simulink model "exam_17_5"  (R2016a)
settings: Solver=ode15s  StartTime=0.0  StopTime=10  RelTol=1e-3
libraries: powerlib x7, dspxfrm3 x2

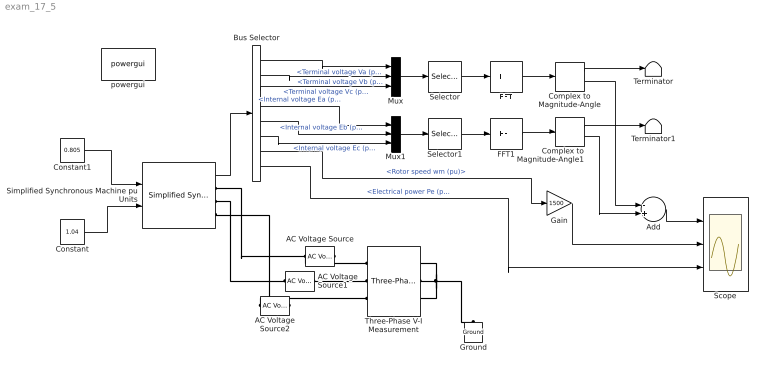
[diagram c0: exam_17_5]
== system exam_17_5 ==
  AC Voltage Source : powerlib/Electrical Sources/AC Voltage Source  Amplitude=10500*1.414/1.732  Phase=0  Frequency=50  SampleTime=0  Measurements=None  BusType=swing  Pref=10e3  Qref=0  Qmin=-inf  Qmax=+inf
  AC Voltage Source1 : powerlib/Electrical Sources/AC Voltage Source  Amplitude=10500*1.414/1.732  Phase=120  Frequency=50  SampleTime=0  Measurements=None  BusType=swing  Pref=10e3  Qref=0  Qmin=-inf  Qmax=+inf
  AC Voltage Source2 : powerlib/Electrical Sources/AC Voltage Source  Amplitude=10500*1.414/1.732  Phase=-120  Frequency=50  SampleTime=0  Measurements=None  BusType=swing  Pref=10e3  Qref=0  Qmin=-inf  Qmax=+inf
  Add : Sum  Inputs=-+
  Bus Selector : BusSelector  OutputSignals=Terminal voltage Va (pu),Terminal voltage Vb (pu),Terminal voltage Vc (pu),Internal voltage Ea (pu),Internal voltage Eb (pu),Internal voltage Ec (pu),Rotor speed wm (pu),Electrical power Pe (pu)
  Complex to Magnitude-Angle : ComplexToMagnitudeAngle
  Complex to Magnitude-Angle1 : ComplexToMagnitudeAngle
  Constant : Constant  Value=1.04  VectorParams1D=off
  Constant1 : Constant  Value=0.805  VectorParams1D=off
  FFT : dspxfrm3/FFT  FFTImplementation=Auto  CompMethod=Table lookup  TableOpt=NEW  TableOptActive=Speed  BitRevOrder=off  Normalize=off  InheritFFTLength=on  FFTLength=64  WrapInput=on  roundingMode=Floor  overflowMode=off  firstCoeffDataTypeStr=Inherit: Same word length as input  firstCoeffLastDataTypeStr=Inherit: Same word length as input  outputMin=[]  outputMax=[]
  FFT1 : dspxfrm3/FFT  FFTImplementation=Auto  CompMethod=Table lookup  TableOpt=NEW  TableOptActive=Speed  BitRevOrder=off  Normalize=off  InheritFFTLength=on  FFTLength=64  WrapInput=on  roundingMode=Floor  overflowMode=off  firstCoeffDataTypeStr=Inherit: Same word length as input  firstCoeffLastDataTypeStr=Inherit: Same word length as input  outputMin=[]  outputMax=[]
  Gain : Gain  Gain=1500
  Ground : powerlib/Elements/Ground  LConnTagsString=a
  Mux : Mux  Inputs=3
  Mux1 : Mux  Inputs=3
  Scope : Scope  NumInputPorts=3
  Selector : Selector  IndexMode=Zero-based  InputPortWidth=3  IndexOptions=Index vector (dialog)  Indices=[0]  OutputSizes=1
  Selector1 : Selector  IndexMode=Zero-based  InputPortWidth=3  IndexOptions=Index vector (dialog)  Indices=[0]  OutputSizes=1
  Simplified Synchronous Machine pu Units : powerlib/Machines/Simplified Synchronous Machine pu Units  ConnectionType=3-wire Y  MechanicalLoad=Mechanical power Pm  MeasurementBus=off  NominalParameters=[50e6 10.5e3 50]  Mechanical=[3 28 2]  InternalRL="[0.005  0.9]"  InitialConditions="[ 0  0  0  0 0  0  0  0 ]"  Units=0  LoadFlowParameters=[1 0 0 0 0]  TsPowergui=0  TsBlock=-1  BusType=swing  Pref=0  Qref=0  Qmin=-inf  Qmax=+inf  PLF=0  QLF=0
  Terminator : Terminator
  Terminator1 : Terminator
  Three-Phase V-I Measurement : powerlib/Measurements/Three-Phase V-I Measurement  VoltageMeasurement=no  SetLabelV=off  LabelV=Vabc  Vpu=off  VpuLL=off  CurrentMeasurement=no  SetLabelI=off  LabelI=Iabc  Ipu=off  Pbase=100e6  Vbase=500e3  OutputType=Complex  PhasorSimulation=off  PSBequivalent=0
  powergui : powerlib/powergui  Priority=1  SimulationMode=Continuous  SolverType=Tustin/Backward Euler (TBE)  SampleTime=50e-6  frequency=60  SPID=on  DisableSnubberDevices=off  DisableRonSwitches=off  DisableVfSwitches=off  SwTol=0  DisplayEquations=off  Interpol=off  ExternalGateDelay=off  methode=off  Ts=10  FunctionMessages=off  echomessages=off  HookPort=off  EnableUseOfTLC=off  x0status=blocks  frequencyindice=50  Pbase=100e6  ErrMax=1e-4  Iterations=50  UnitsV=kV  UnitsW=MW  buscounter=0  RestoreLinks=warning  ResistiveCurrentMeasurement=off  Frange=[0:2:500]  Ylog=off  Xlog=on  ShowGrid=off  save=off  variable=ZData  structure=0  ZoomFFT=off  StartTime=0.0  cycles=1  DisplayStyle=1  fundamental=60  FreqAxis=off  MaxFrequency=1000  frequencyindicesteady=1  RmsSteady=1  display=off
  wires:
  Constant/1 -> Simplified Synchronous Machine pu Units/2
  Complex to Magnitude-Angle/1 -> Terminator/1
  Complex to Magnitude-Angle1/1 -> Terminator1/1
  Complex to Magnitude-Angle1/2 -> Add/2
  Add/1 -> Scope/1
  Gain/1 -> Scope/2
  Mux/1 -> Selector/1
  Mux1/1 -> Selector1/1
  Simplified Synchronous Machine pu Units/1 -> Bus Selector/1
  Bus Selector/1 -> Mux/1  "<Terminal voltage Va (pu)>"
  Bus Selector/2 -> Mux/2  "<Terminal voltage Vb (pu)>"
  Bus Selector/3 -> Mux/3  "<Terminal voltage Vc (pu)>"
  Bus Selector/4 -> Mux1/1  "<Internal voltage Ea (pu)>"
  Bus Selector/5 -> Mux1/2  "<Internal voltage Eb (pu)>"
  Bus Selector/6 -> Mux1/3  "<Internal voltage Ec (pu)>"
  Bus Selector/7 -> Gain/1  "<Rotor speed wm (pu)>"
  Complex to Magnitude-Angle/2 -> Add/1
  Constant1/1 -> Simplified Synchronous Machine pu Units/1
  Bus Selector/8 -> Scope/3  "<Electrical power Pe (pu)>"
  Selector/1 -> FFT/1
  Selector1/1 -> FFT1/1
  FFT1/1 -> Complex to Magnitude-Angle1/1
  FFT/1 -> Complex to Magnitude-Angle/1
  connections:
  Simplified Synchronous Machine pu Units/RConn1 -- AC Voltage Source/RConn1
  AC Voltage Source/LConn1 -- Three-Phase V-I Measurement/LConn1
  Simplified Synchronous Machine pu Units/RConn2 -- AC Voltage Source1/RConn1
  AC Voltage Source1/LConn1 -- Three-Phase V-I Measurement/LConn2
  AC Voltage Source2/RConn1 -- Simplified Synchronous Machine pu Units/RConn3
  AC Voltage Source2/LConn1 -- Three-Phase V-I Measurement/LConn3
  Three-Phase V-I Measurement/RConn2 -- Three-Phase V-I Measurement/RConn3 -- Three-Phase V-I Measurement/RConn1 -- Ground/LConn1
